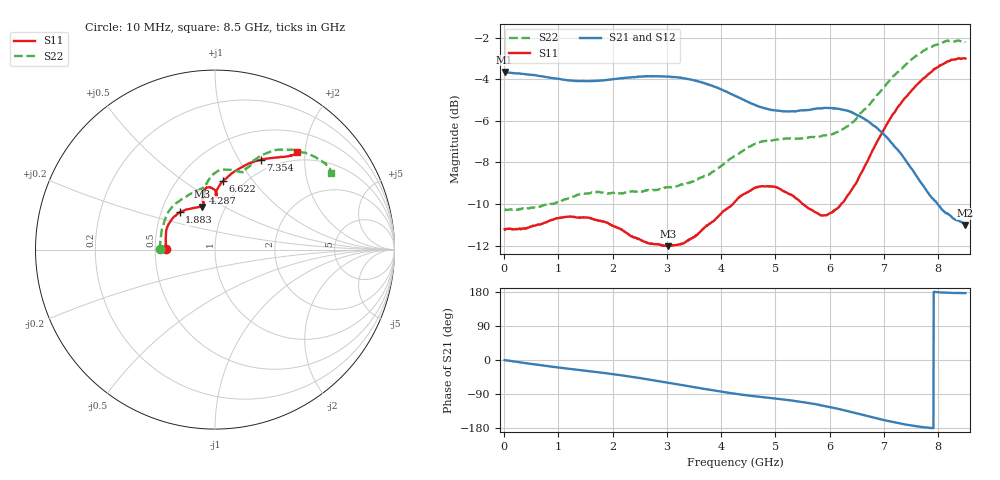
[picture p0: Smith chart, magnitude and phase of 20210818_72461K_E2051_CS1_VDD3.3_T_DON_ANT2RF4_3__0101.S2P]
!Agilent Technologies,E5071C,MY46417908,A.11.23
!Date: Wed Aug 18 14:34:04 2021
!Data & Calibration Information:
!Freq	S11:SOLT2(ON)	S21:SOLT2(ON)	S12:SOLT2(ON)	S22:SOLT2(ON)
!PortZ  Port1:50+j0  Port2:50+j0
!Above PortZ is port z conversion or system Z0 setting when saving the data.
!When reading, reference impedance value at option line is always used.
# Hz S dB R 50
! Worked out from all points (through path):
!   1601 points, 10 MHz to 8.5 GHz, reference 50 ohm
!   highest |S21| = -3.65 dB at 10 MHz (marker M1); lowest = -11.0 dB at 8.5 GHz (marker M2)
!   group delay of S21, straight-line fit = 63.3 ps
!   lowest |S11| = -12.0 dB at 3.019 GHz (marker M3), VSWR 1.67, Z = 38.7 + j19.8 ohm
!   |S11| at or under -10 dB: start of sweep to 4.217 GHz; 5.5 GHz to 6.212 GHz (711.3 MHz wide, 12.1 % of centre)
!   |S22| runs from -10.3 to -2.1 dB; largest |S21 - S12| = 0.0017
!   S11 on the Smith chart (normalised r, x): 10 MHz: 0.57, +0.00; 1.883 GHz: 0.62, +0.28; 4.287 GHz: 0.73, +0.51; 6.622 GHz: 0.81, +0.72; 7.354 GHz: 0.85, +1.24; 8.5 GHz: 0.84, +1.83
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1e7  -11.21 179.6  -3.65 -0.4  -3.65 -0.3  -10.25 179.8
9.492062e8  -10.70 158.8  -3.96 -18.9  -3.95 -18.9  -9.95 155.3
1.426769e9  -10.65 146.1  -4.09 -27.1  -4.09 -27.0  -9.51 140.6
1.883106e9  -10.88 133.5  -4.03 -35.0  -4.03 -35.0  -9.48 127.0
2.334138e9  -11.55 120.8  -3.91 -44.1  -3.92 -44.1  -9.41 114.7
2.843538e9  -11.94 109.6  -3.85 -55.6  -3.85 -55.7  -9.31 104.9
3.018644e9  -12.03 107.1  -3.87 -59.8  -3.86 -59.8  -9.19 103.1
3.61825e9  -11.32 103.7  -4.13 -74.5  -4.12 -74.5  -8.72 98.0
4.255e9  -9.89 101.6  -4.79 -88.9  -4.78 -88.9  -7.68 92.5
4.286838e9  -9.80 101.4  -4.83 -89.6  -4.83 -89.6  -7.64 92.2
4.631744e9  -9.21 98.6  -5.24 -95.9  -5.24 -95.9  -7.10 87.2
4.97665e9  -9.17 94.3  -5.49 -101.4  -5.49 -101.3  -6.92 80.8
5.671769e9  -10.29 88.4  -5.45 -114.9  -5.46 -114.9  -6.78 70.8
5.899938e9  -10.53 88.6  -5.38 -121.1  -5.39 -121.1  -6.70 69.4
6.138719e9  -10.22 89.5  -5.42 -128.4  -5.43 -128.5  -6.54 69.2
6.621588e9  -8.31 83.3  -5.88 -145.3  -5.87 -145.4  -5.50 67.2
7.088538e9  -6.00 70.1  -6.90 -161.5  -6.91 -161.6  -4.10 60.7
7.35385e9  -5.01 62.9  -7.74 -169.2  -7.73 -169.2  -3.42 55.5
7.587325e9  -4.31 57.2  -8.61 -174.7  -8.60 -174.8  -2.88 50.4
7.937538e9  -3.49 51.4  -9.84 179.6  -9.83 179.6  -2.36 42.2
8.139175e9  -3.20 49.9  -10.44 177.7  -10.41 177.7  -2.18 38.2
8.5e9  -3.00 50.0  -11.01 176.5  -10.99 176.4  -2.22 33.6
